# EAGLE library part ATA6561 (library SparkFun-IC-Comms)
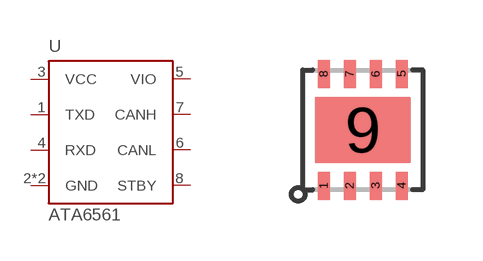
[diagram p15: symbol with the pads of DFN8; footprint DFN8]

Designator prefix U

## ATA6561 (PROD_ID: IC-13837)  [DFN8]
1  TXD
2  GND
3  VCC
4  RXD
5  VIO
6  CANL
7  CANH
8  STBY
9  GND

## Footprint DFN8 (pad centres in mm)
smd 0.3 x 0.7: 1 -0.975,-1.4; 2 -0.325,-1.4; 3 0.325,-1.4; 4 0.975,-1.4; 5 0.975,1.4; 6 0.325,1.4; 7 -0.325,1.4; 8 -0.975,1.4
smd 2.38 x 1.65: 9 0,0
